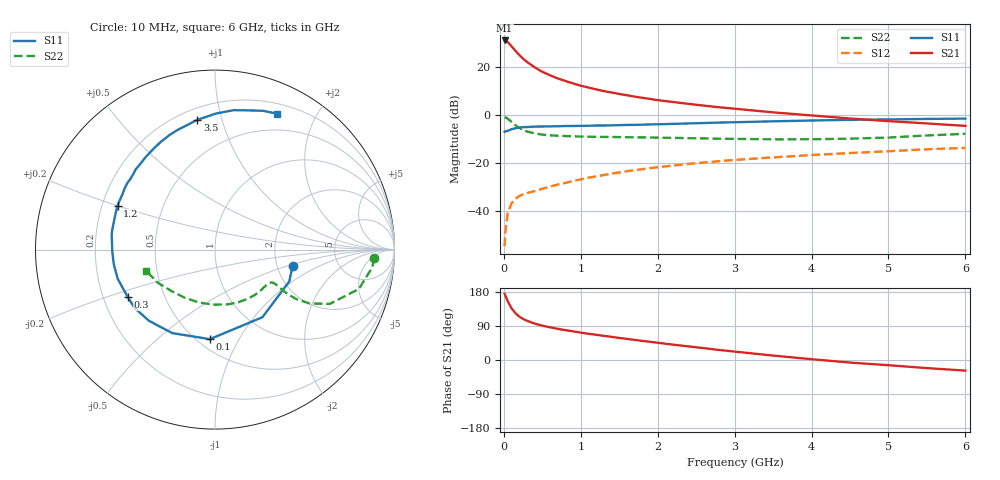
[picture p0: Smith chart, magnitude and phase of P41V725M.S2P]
! SIEMENS Small Signal Semiconductors
! BFP182
! Si NPN RF Bipolar Junction Transistor in SOT143
! VCE = 1.75 V  IC = 25 mA
! Common Emitter S-Parameters:  March  1996
# GHz  S  MA  R  50
!  f  S11  S21  S12  S22
! GHz  MAG  ANG  MAG  ANG  MAG  ANG  MAG  ANG
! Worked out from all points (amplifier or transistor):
!   36 points, 10 MHz to 6 GHz, reference 50 ohm
!   highest |S21| = 31.0 dB at 10 MHz (marker M1)
!   |S21| within 3 dB of that: start of sweep to 114.9 MHz
!   unconditionally stable (mu >= 1): start of sweep to 14.08 MHz; 375 MHz to end of sweep
!   at 250 MHz: K = 0.76, MSG = 28.3 dB, |S12| = -33.3 dB
!   at 1.4 GHz: K = 1.52, MAG = 12.7 dB, |S12| = -24.6 dB
!   at 6 GHz: K = 1.12, MAG = 2.5 dB, |S12| = -13.9 dB
!   S11 on the Smith chart (normalised r, x): 10 MHz: 2.44, -0.55; 100 MHz: 0.57, -0.76; 300 MHz: 0.30, -0.23; 1.2 GHz: 0.26, +0.20; 3.5 GHz: 0.27, +0.84; 6 GHz: 0.31, +1.51
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0.01  0.442 -11.9  35.65 174.8  0.0018 77.1  0.8888 -3.0
0.02  0.4501 -23.3  35.56 169.9  0.0036 75.2  0.882 -6.4
0.05  0.4602 -55.0  33.18 155.2  0.0088 71.9  0.8313 -15.3
0.1  0.4997 -93.3  26.9 136.4  0.0141 57.2  0.7075 -25.3
0.15  0.5227 -117.1  21.72 123.6  0.0175 50.5  0.6057 -29.7
0.2  0.5412 -132.9  17.76 114.7  0.02 48.3  0.5321 -31.3
0.25  0.5532 -143.9  14.81 108.3  0.0217 46.3  0.4817 -31.5
0.3  0.5533 -151.6  12.74 103.7  0.0231 46.9  0.4488 -31.1
0.4  0.566 -163.3  9.826 96.1  0.0254 48.1  0.4083 -30.2
0.5  0.5698 -171.7  7.901 90.7  0.0285 49.5  0.3853 -29.7
0.6  0.5721 -178.5  6.684 86.2  0.0316 52.0  0.3726 -29.7
0.7  0.5751 176.2  5.73 82.3  0.0348 53.5  0.3643 -30.2
0.8  0.5826 171.3  5.067 78.7  0.0377 54.7  0.3588 -31.0
1.1  0.5902 159.4  3.699 69.2  0.0485 55.8  0.3482 -34.7
1.2  0.5955 155.8  3.388 66.6  0.0515 55.7  0.3461 -36.3
1.7  0.6146 139.8  2.393 53.0  0.0696 54.7  0.3379 -45.3
2.2  0.6447 126.6  1.848 40.5  0.087 51.5  0.3301 -56.2
2.8  0.6868 111.6  1.434 26.4  0.1073 46.4  0.3157 -71.2
3.5  0.7296 97.8  1.123 11.7  0.1287 40.2  0.3069 -91.4
4.5  0.7836 82.4  0.836 -6.8  0.1586 31.3  0.3169 -122.5
5.5  0.8183 70.9  0.659 -21.4  0.1903 22.1  0.3693 -150.2
6  0.8323 65.5  0.586 -28.0  0.203 16.7  0.4005 -162.8
